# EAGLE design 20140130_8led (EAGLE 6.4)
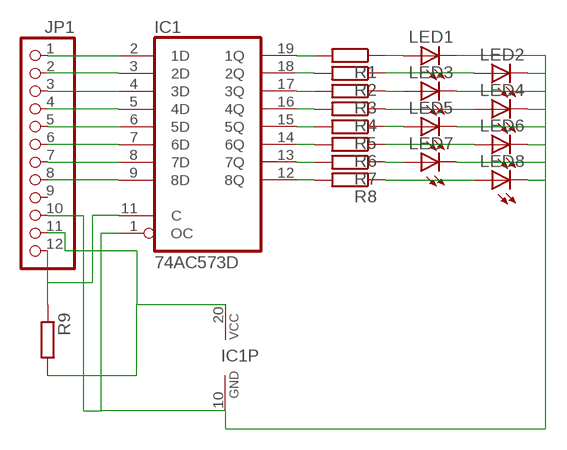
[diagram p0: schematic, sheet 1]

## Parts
IC1  74AC573D  [SO20W]
JP1  PINHD-1X12  [1X12]
LED1  LEDCHIPLED_1206  [CHIPLED_1206]
LED2  LEDCHIPLED_1206  [CHIPLED_1206]
LED3  LEDCHIPLED_1206  [CHIPLED_1206]
LED4  LEDCHIPLED_1206  [CHIPLED_1206]
LED5  LEDCHIPLED_1206  [CHIPLED_1206]
LED6  LEDCHIPLED_1206  [CHIPLED_1206]
LED7  LEDCHIPLED_1206  [CHIPLED_1206]
LED8  LEDCHIPLED_1206  [CHIPLED_1206]
R1  R-EU_R1206  [R1206]
R2  R-EU_R1206  [R1206]
R3  R-EU_R1206  [R1206]
R4  R-EU_R1206  [R1206]
R5  R-EU_R1206  [R1206]
R6  R-EU_R1206  [R1206]
R7  R-EU_R1206  [R1206]
R8  R-EU_R1206  [R1206]
R9  R-EU_R1206  [R1206]

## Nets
GND: IC1.1(OC) IC1.10(GND) JP1.10 LED1.C LED2.C LED3.C LED4.C LED5.C LED6.C LED7.C LED8.C
N$1: IC1.2(1D) JP1.1
N$2: IC1.3(2D) JP1.2
N$3: IC1.4(3D) JP1.3
N$4: IC1.5(4D) JP1.4
N$5: IC1.6(5D) JP1.5
N$6: IC1.7(6D) JP1.6
N$7: IC1.8(7D) JP1.7
N$8: IC1.9(8D) JP1.8
N$12: LED8.A R8.1
N$13: LED6.A R6.1
N$14: LED7.A R7.1
N$15: LED5.A R5.1
N$16: LED4.A R4.1
N$17: LED2.A R2.1
N$18: LED3.A R3.1
N$19: LED1.A R1.1
N$20: IC1.19(1Q) R1.2
N$21: IC1.18(2Q) R2.2
N$22: IC1.17(3Q) R3.2
N$23: IC1.16(4Q) R4.2
N$24: IC1.15(5Q) R5.2
N$25: IC1.14(6Q) R6.2
N$26: IC1.13(7Q) R7.2
N$27: IC1.12(8Q) R8.2
N$29: IC1.11(C) JP1.12 R9.1
VCC: IC1.20(VCC) JP1.11 R9.2
Unconnected: JP1.9

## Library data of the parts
IC1 = 74xx-eu:74*573: 8-bit D latch BUS DRIVER
JP1 = pinhead:PINHD-1X12: PIN HEADER
LED1-LED8 = led:LED: LED
R1-R9 = rcl:R-EU_: RESISTOR, European symbol

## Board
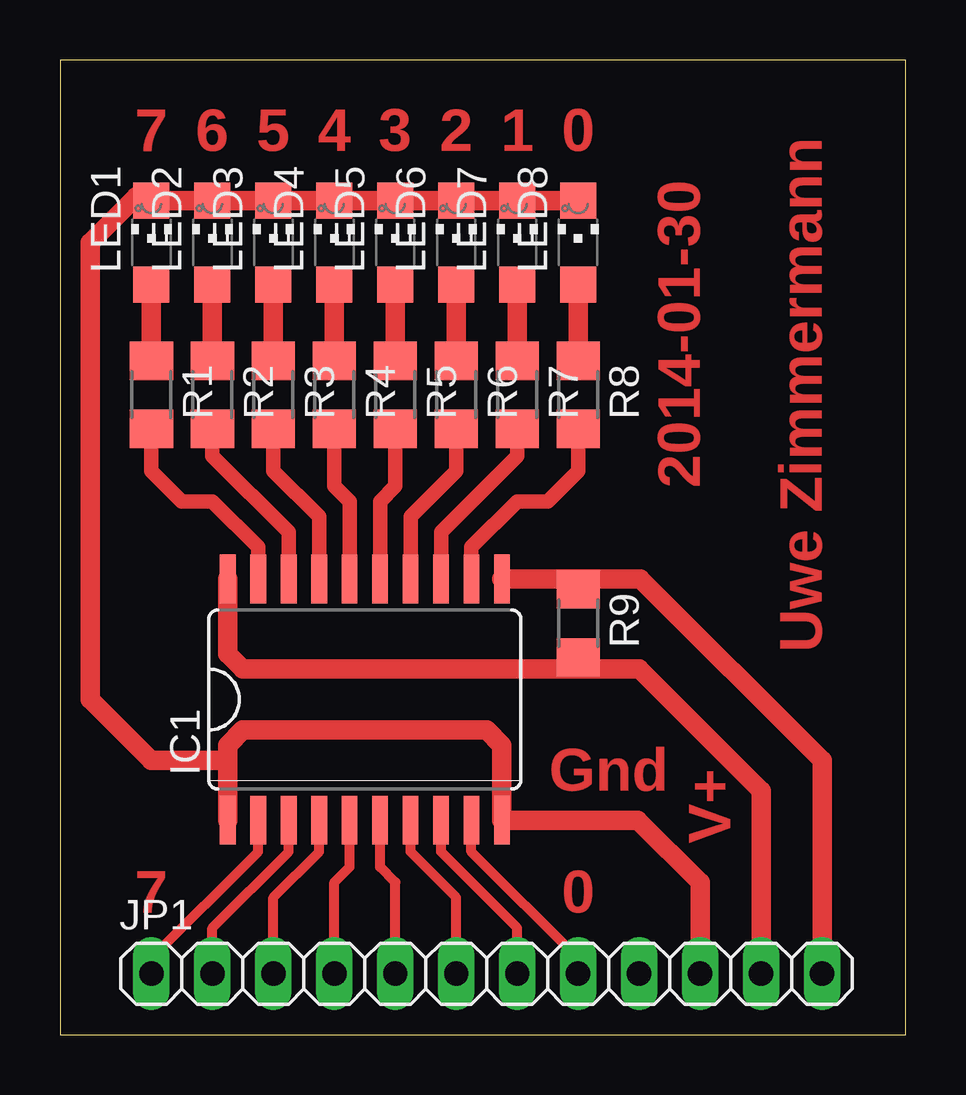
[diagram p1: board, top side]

Size 35.23 x 40.63 mm. Coordinates in mm from the lower left corner, seen from the top.
Outline: 0,0 35.23,0 35.23,40.63 0,40.63 0,0
Copper layers (1*16): Top 0.035mm / dielectric 1.5mm / Bottom 0.035mm
Design rules "default": minimum track width 10mil, minimum drill 24mil, track to track 8mil, track to pad 8mil, pad to pad 8mil, via to via 8mil, smd to smd 8mil, copper to edge 40mil, drill to drill 8mil, minimum pad ring 10mil, minimum via ring 8mil, stop-mask expansion 4mil, vias tented up to drill 0mil, thermal gap 10mil

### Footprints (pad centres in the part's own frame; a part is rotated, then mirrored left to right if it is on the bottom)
SO20W = smd 0.66 x 2.032: 1 -5.715,-5.029; 2 -4.445,-5.029; 3 -3.175,-5.029; 4 -1.905,-5.029; 5 -0.635,-5.029; 6 0.635,-5.029; 7 1.905,-5.029; 8 3.175,-5.029; 9 4.445,-5.029; 10 5.715,-5.029; 11 5.715,5.029; 12 4.445,5.029; 13 3.175,5.029; 14 1.905,5.029; 15 0.635,5.029; 16 -0.635,5.029; 17 -1.905,5.029; 18 -3.175,5.029; 19 -4.445,5.029; 20 -5.715,5.029
1X12 = drill 1.016 long: 1 -13.97,0; 2 -11.43,0; 3 -8.89,0; 4 -6.35,0; 5 -3.81,0; 6 -1.27,0; 7 1.27,0; 8 3.81,0; 9 6.35,0; 10 8.89,0; 11 11.43,0; 12 13.97,0
CHIPLED_1206 = smd 1.5 x 1.5: A 0,-1.75; C 0,1.75
R1206 = smd 1.6 x 1.803: 1 -1.422,0; 2 1.422,0

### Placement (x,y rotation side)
IC1  12.7,13.97 0 top
JP1  17.78,2.54 0 top
LED1  3.81,33.02 0 top
LED2  6.35,33.02 0 top
LED3  8.89,33.02 0 top
LED4  11.43,33.02 0 top
LED5  13.97,33.02 0 top
LED6  16.51,33.02 0 top
LED7  19.05,33.02 0 top
LED8  21.59,33.02 0 top
R1  3.81,26.67 270 top
R2  6.35,26.67 270 top
R3  8.89,26.67 270 top
R4  11.43,26.67 270 top
R5  13.97,26.67 270 top
R6  16.51,26.67 270 top
R7  19.05,26.67 270 top
R8  21.59,26.67 270 top
R9  21.59,17.14 270 top

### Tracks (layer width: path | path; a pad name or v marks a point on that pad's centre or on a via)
GND
  Top 0.813: IC1.1 6.99,11.43 | 6.99,11.43 6.99,12.06 7.62,12.7 17.78,12.7 18.41,12.06 IC1.10 24.08,8.94 26.67,6.35 JP1.10 | LED8.C LED7.C LED6.C LED5.C LED4.C LED3.C LED2.C LED1.C 3.65,34.92 3.17,34.92 1.27,33.02 1.27,13.97 3.81,11.43 6.99,11.43
N$1
  Top 0.406: JP1.1 3.81,3.17 8.26,7.62 IC1.2
N$2
  Top 0.406: JP1.2 6.35,4.45 9.53,7.62 IC1.3
N$3
  Top 0.406: JP1.3 8.89,5.71 10.79,7.62 IC1.4
N$4
  Top 0.406: JP1.4 11.43,6.35 12.06,6.99 IC1.5
N$5
  Top 0.406: JP1.5 13.97,6.35 13.34,6.99 IC1.6
N$6
  Top 0.406: JP1.6 16.51,5.71 14.61,7.62 IC1.7
N$7
  Top 0.406: JP1.7 19.05,4.45 15.88,7.62 IC1.8
N$8
  Top 0.406: JP1.8 21.59,3.17 17.14,7.62 IC1.9
N$12
  Top 0.813: LED8.A R8.1
N$13
  Top 0.813: LED6.A R6.1
N$14
  Top 0.813: LED7.A R7.1
N$15
  Top 0.813: LED5.A R5.1
N$16
  Top 0.813: LED4.A R4.1
N$17
  Top 0.813: LED2.A R2.1
N$18
  Top 0.813: LED3.A R3.1
N$19
  Top 0.813: LED1.A R1.1
N$20
  Top 0.61: IC1.19 8.26,20.32 6.35,22.23 5.08,22.23 3.81,23.5 R1.2
N$21
  Top 0.61: IC1.18 9.53,20.95 6.35,24.13 R2.2
N$22
  Top 0.61: IC1.17 10.79,21.59 8.89,23.5 R3.2
N$23
  Top 0.61: IC1.16 12.06,22.23 11.43,22.86 R4.2
N$24
  Top 0.61: IC1.15 13.34,22.23 13.97,22.86 R5.2
N$25
  Top 0.61: IC1.14 14.61,21.59 16.51,23.5 R6.2
N$26
  Top 0.61: IC1.13 15.88,20.95 19.05,24.13 R7.2
N$27
  Top 0.61: IC1.12 17.14,20.32 19.05,22.23 20.32,22.23 21.59,23.5 R8.2
N$29
  Top 0.813: JP1.12 31.75,11.43 24.18,19 IC1.11 21.16,19 R9.1
VCC
  Top 0.813: IC1.20 6.99,15.88 7.62,15.24 21.59,15.24 | 21.59,15.24 24.13,15.24 29.21,10.16 JP1.11 | R9.2 21.59,15.24

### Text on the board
Top: 7 | 6 | 5 | 4 | 3 | 2 | 1 | 0 | 2014-01-30 | Uwe Zimmermann | Gnd | V+ | 7 | 0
